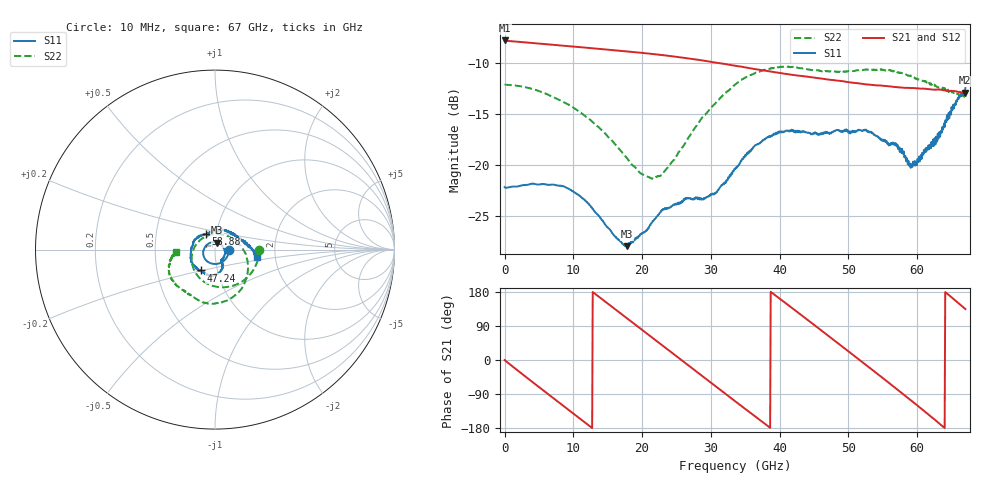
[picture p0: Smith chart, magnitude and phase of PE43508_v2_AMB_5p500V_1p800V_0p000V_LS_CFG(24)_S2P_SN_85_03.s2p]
!Keysight Technologies,N5227A,US51270237,A.10.43.00
!Date: Wednesday, August 22, 2018 17:09:02
!Correction: S11(Full 2 Port(1,3))
!S31(Full 2 Port(1,3))
!S13(Full 2 Port(1,3))
!S33(Full 2 Port(1,3))
!S2P File: Measurements: S11, S31, S13, S33:
# Hz S  dB  R 50
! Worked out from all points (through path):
!   801 points, 10 MHz to 67 GHz, reference 50 ohm
!   highest |S21| = -7.81 dB at 10 MHz (marker M1); lowest = -12.9 dB at 66.92 GHz (marker M2)
!   group delay of S21, straight-line fit = 38.8 ps
!   lowest |S11| = -28.0 dB at 17.76 GHz (marker M3), VSWR 1.08, Z = 50.8 + j3.93 ohm
!   |S11| at or under -10 dB: start of sweep to end of sweep
!   |S22| runs from -21.4 to -10.3 dB; largest |S21 - S12| = 0.0022
!   S11 on the Smith chart (normalised r, x): 10 MHz: 1.17, -0.00; 47.24 GHz: 0.83, -0.20; 58.88 GHz: 0.89, +0.15; 67 GHz: 1.60, -0.14
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1e7  -22.20 -0.6  -7.81 -0.2  -7.81 -0.2  -12.12 -0.3
2.522125e9  -22.03 -41.3  -7.97 -36.4  -7.96 -36.4  -12.33 -28.8
5.70415e9  -21.90 -88.4  -8.15 -81.3  -8.14 -81.3  -12.94 -63.3
8.300012e9  -22.08 -124.2  -8.31 -117.7  -8.30 -117.6  -13.77 -90.5
1.123082e10  -23.24 -162.9  -8.48 -158.5  -8.48 -158.5  -14.95 -120.3
1.424538e10  -25.46 151.2  -8.66 159.6  -8.66 159.6  -16.69 -152.2
1.776235e10  -28.00 76.0  -8.88 110.8  -8.88 110.7  -19.31 163.5
2.002326e10  -26.75 27.3  -9.03 79.2  -9.03 79.2  -20.93 126.0
2.236791e10  -24.91 -13.1  -9.20 46.6  -9.21 46.6  -21.15 81.4
2.471256e10  -23.92 -38.7  -9.39 13.8  -9.39 13.9  -19.48 41.2
2.705721e10  -23.35 -53.6  -9.61 -18.9  -9.60 -18.7  -17.03 10.3
3.040671e10  -22.93 -59.5  -9.95 -65.5  -9.94 -65.4  -14.13 -21.8
3.3505e10  -20.42 -64.3  -10.28 -108.5  -10.27 -108.4  -12.15 -47.6
3.88642e10  -17.22 -89.3  -10.87 177.6  -10.88 177.7  -10.55 -84.2
4.472582e10  -16.96 -116.9  -11.42 96.6  -11.41 96.6  -10.72 -113.5
4.723795e10  -16.99 -124.8  -11.66 61.5  -11.65 61.3  -10.87 -121.5
5.150856e10  -16.56 -145.5  -12.02 1.5  -12.01 1.5  -10.73 -133.3
5.586291e10  -18.12 167.7  -12.30 -60.1  -12.31 -60.4  -10.72 -149.6
5.887746e10  -20.08 120.8  -12.47 -103.4  -12.48 -103.6  -11.29 -160.2
6.314808e10  -17.27 35.5  -12.63 -166.6  -12.67 -166.8  -12.45 -171.0
6.691626e10  -12.94 -8.7  -12.93 135.8  -12.99 135.9  -13.14 -175.7
6.7e10  -12.48 -10.1  -12.92 134.4  -12.98 134.5  -13.22 -176.7
